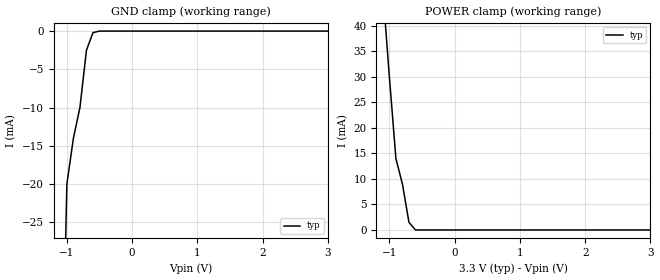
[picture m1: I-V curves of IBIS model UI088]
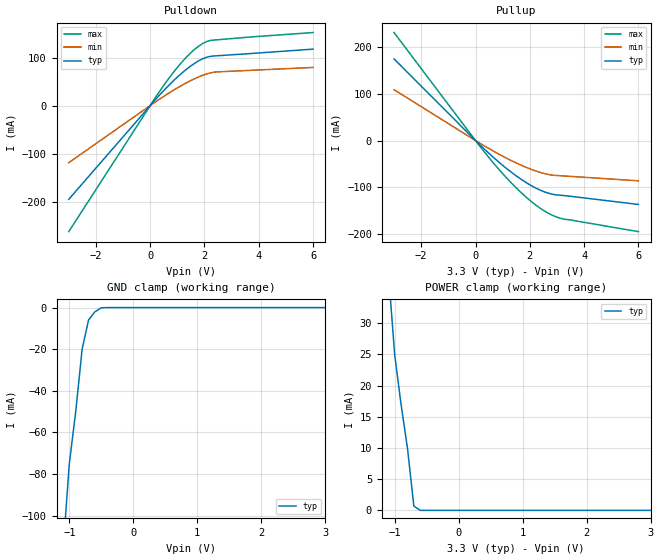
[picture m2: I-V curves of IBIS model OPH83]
|   TEXAS INSTRUMENTS INCORPORATION
|   IBIS MODEL OF SN74V245(PAG64)
[IBIS Ver]   2.1
[File Name]   sn74v245.ibs
[File Rev]   0.1
[Date]   Mon Dec 25 15:22:22 JST 2000
[Source]   IBIS Model Generated from PACED 4.40B
[Disclaimer]   Please be aware that in the absence of a written agreement
|   Texas Instruments(TI) assumes no liability for:
|   (1) The accuracy of the IBIS models provided to your company
|   (2) The proper functioning of these Models in your design
|   or for any resulting applications;or
|   (3)Infringement of patents,copyrights or intellectual
|   property rights resulting from your use of these models.
|   TI provides IBIS Models as a service to our customers and
|   therefore reserves the right to limit distribution of the
|   Models.
[Copyright]   Property of Texas Instruments Incorporated.
|   Unauthorised reproduction and/or distribution is strictly
|   prohibited.
|   This product is protected under copyright law and trade
|   secret law as an unpublished work.
|   Created 1999,(C) Copyright 1999-2000,
|   Texas Instruments Incorporated., All Rights Reserved.
|   These commodities are under the U.S.
|   Government distribution license control.As such,they are not
|   to be re-exported without the prior approval of the U.S.
|   Department of Commerce.
[component]   SN74V245
[Manufacturer]   Texas Instruments Inc.
[Package]
| Variable   Typ   Min   Max
R_pkg   0.05841   0.05659   0.06088
L_pkg   2.698e-09   2.631e-09   2.866e-09
C_pkg   4.671e-13   3.884e-13   5.134e-13
[Pin]   signal_name  model_name  R_pin   L_pin   C_pin
1   A   UI088   0.05717   2.859e-09   4.649e-13
49   VCC   POWER   0.05717   2.859e-09   4.649e-13
50   Y   OPH83   0.05659   2.744e-09   5.134e-13
51   GND   GND   0.0566   2.696e-09   5.033e-13
| Models and submodels in the file (2): UI088 (Input), OPH83 (3-state)
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[Model]   UI088
Model_type   Input
Polarity   Non-Inverting
| signals   A, Y
Vinl = 0.8V
Vinh = 2.0V
|   typ   min   max
C_comp   1.001p   0.989p   1.023p
|   typ   min   max
[Temperature Range]   25.0   0   115
|   typ   min   max
[Voltage Range]   3.3V   3.0V   3.6V
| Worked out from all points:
|   GND clamp passes 1 mA (typ) near -0.63 V on its own axis
|   POWER clamp passes 1 mA (typ) near -0.67 V on its own axis
[GND_clamp]
|   Voltage   I(typ)   I(min)   I(max)
-3V       -900mA     NA         NA
-2V       -400mA     NA         NA
-1V       -20mA      NA         NA
-900mV    -14mA      NA         NA
-800mV    -10mA      NA         NA
-700mV    -2.5mA     NA         NA
-600mV    -200uA     NA         NA
-500mV    0A         NA         NA
3V        0A         NA         NA
[POWER_clamp]
|   Voltage   I(typ)   I(min)   I(max)
-3V       600mA      NA         NA
-2V       200mA      NA         NA
-1V       30mA       NA         NA
-900mV    14mA       NA         NA
-800mV    9mA        NA         NA
-700mV    1.5mA      NA         NA
-600mV    0A         NA         NA
-500mV    0A         NA         NA
3V        0A         NA         NA
[Model]   OPH83
Model_type   3-state
Polarity   Non-Inverting
Enable   Active-Low
| signals   A, GZ, Y
Rref = 50
Vmeas = 1.3
|   typ   min   max
C_comp   1.634p   1.612p   1.687p
|   typ   min   max
[Temperature Range]   25.0   0   115
|   typ   min   max
[Voltage Range]   3.3V   3.0V   3.6V
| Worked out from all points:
|   slope of the pulldown table from 0 to 0.495 V, typ, clamps not added: 16 ohm
|   slope of the pullup table from 0 to 0.495 V, typ, clamps not added: 18 ohm
|   GND clamp passes 1 mA (typ) near -0.55 V on its own axis
|   POWER clamp passes 1 mA (typ) near -0.70 V on its own axis
[Pulldown]
|   Voltage   I(typ)   I(min)   I(max)
-3V       -195.2mA   -118.9mA   -262.4mA
400mV     25.31mA    15.47mA    34mA
800mV     48.5mA     29.9mA     65.01mA
1.1V      64.32mA    39.99mA    86mA
1.4V      78.4mA     49.28mA    104.5mA
1.7V      90.23mA    57.53mA    119.9mA
2V        98.96mA    64.34mA    131.1mA
2.3V      103mA      69mA       136.1mA
6V        117.5mA    79.33mA    152mA
[GND_clamp]
|   Voltage   I(typ)   I(min)   I(max)
-3V       -900mA     NA         NA
-2V       -500mA     NA         NA
-1V       -75mA      NA         NA
-900mV    -50mA      NA         NA
-800mV    -20mA      NA         NA
-700mV    -6mA       NA         NA
-600mV    -2mA       NA         NA
-500mV    -120uA     NA         NA
-400mV    0A         NA         NA
3V        0A         NA         NA
[Pullup]
|   Voltage   I(typ)   I(min)   I(max)
-3V       175.2mA    109.2mA    231.9mA
400mV     -22.42mA   -14.04mA   -29.81mA
1.2V      -62.7mA    -39.63mA   -83.76mA
1.6V      -80.07mA   -50.9mA    -107.4mA
2V        -95.05mA   -60.77mA   -128.4mA
2.6V      -111.5mA   -71.83mA   -153.4mA
3.1V      -117.3mA   -75.53mA   -166.6mA
6V        -137.3mA   -86.56mA   -195.7mA
[POWER_clamp]
|   Voltage   I(typ)   I(min)   I(max)
-3V       300mA      NA         NA
-2V       160mA      NA         NA
-1V       25mA       NA         NA
-900mV    17mA       NA         NA
-800mV    10mA       NA         NA
-700mV    700uA      NA         NA
-600mV    0A         NA         NA
-500mV    0A         NA         NA
3V        0A         NA         NA
[Ramp]
|   I(typ)   I(min)   I(max)
dV/dt_r   1.488/0.110n   1.300/0.140n   1.577/0.090n
dV/dt_f   1.443/0.150n   1.260/0.210n   1.534/0.120n
